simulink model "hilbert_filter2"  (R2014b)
settings: Solver=ode45  StartTime=0.0  StopTime=10.0  RelTol=1e-3
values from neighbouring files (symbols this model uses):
  delta = nord/2    (= 32)    [hilbert_filter_1.m]    (also in hilbert_filter_2.m; hilbert_filter_3.m; inv_sinc_1.m = 25; komplexe_huelle_1.m)
  hd = Hd.numerator    [fdesign_1.m]    (also in grp_komp_1.m = fdesign.lowpass('N,Fp,Ap,Ast',nord,fr,dp,ds); hilbert_filter_1.m = design(d, 'equiripple'); hilbert_filter_2.m = design(d, 'equiripple'); hilbert_filter_3.m = design(d, 'equiripple'))
  Ts = 1/fs    (= 0.001)    [abtast_fir_1.m]    (also in abtast_fir_2.m; abtast_fir_3.m; abtast_fir_4.m; hilbert_filter_1.m)
libraries: dspstat3 x2, dsparch4 x1

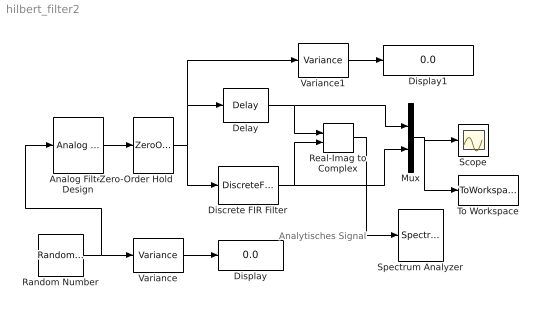
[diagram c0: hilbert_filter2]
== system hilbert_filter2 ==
  note: Analytisches Signal
  Analog Filter Design : dsparch4/Analog Filter Design  method=Elliptic  filttype=Bandpass  N=8  Wlo=2*pi*100  Whi=2*pi*300  Rp=2  Rs=40
  Delay : Delay  DelayLength=delta  UseCircularBuffer=on  SampleTime=Ts
  Discrete FIR Filter : DiscreteFir  Coefficients=hd.numerator
  Display : Display
  Display1 : Display
  Mux : Mux  Inputs=2
  Random Number : RandomNumber  SampleTime=Ts/10
  Real-Imag to Complex : RealImagToComplex
  Scope : Scope
  Spectrum Analyzer : SpectrumAnalyzer
  To Workspace : ToWorkspace  VariableName=y  SaveFormat=Timeseries  SampleTime=-1
  Variance : dspstat3/Variance  run=on  reset_popup=None  InputProcessing=Columns as channels (frame based)  directionMode=Each column  dimension=1  treatSBRowAsCol=on  roiEnable=off  roiType=Rectangles  roiPortion=Entire ROI  roiOutput=Individual statistics for each ROI  roiFlag=off  roundingMode=Floor  overflowMode=off
  Variance1 : dspstat3/Variance  run=on  reset_popup=None  InputProcessing=Columns as channels (frame based)  directionMode=Each column  dimension=1  treatSBRowAsCol=on  roiEnable=off  roiType=Rectangles  roiPortion=Entire ROI  roiOutput=Individual statistics for each ROI  roiFlag=off  roundingMode=Floor  overflowMode=off
  Zero-Order Hold : ZeroOrderHold  SampleTime=Ts
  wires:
  Analog Filter Design/1 -> Zero-Order Hold/1
  Mux/1 -> To Workspace/1, Scope/1
  Discrete FIR Filter/1 -> Mux/2, Real-Imag to Complex/2
  Zero-Order Hold/1 -> Discrete FIR Filter/1, Variance1/1, Delay/1
  Delay/1 -> Mux/1, Real-Imag to Complex/1
  Variance/1 -> Display/1
  Variance1/1 -> Display1/1
  Random Number/1 -> Analog Filter Design/1, Variance/1
  Real-Imag to Complex/1 -> Spectrum Analyzer/1
